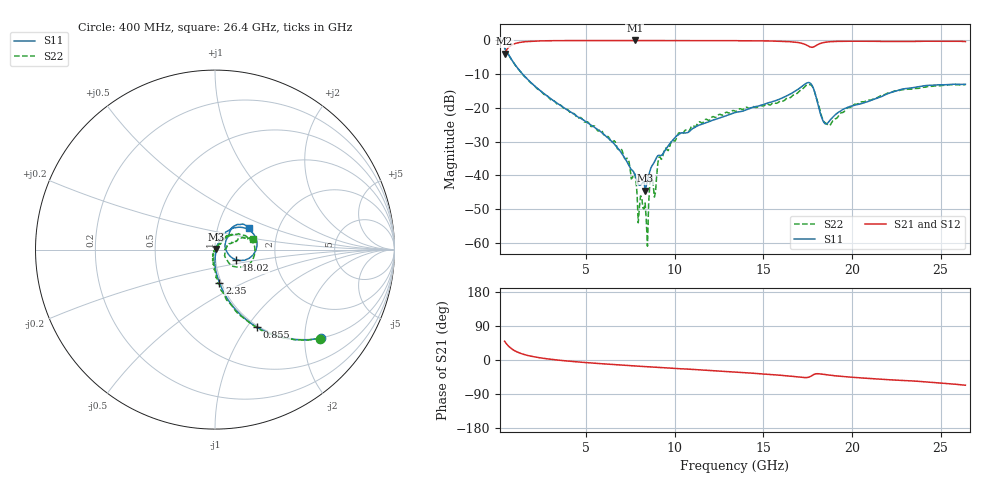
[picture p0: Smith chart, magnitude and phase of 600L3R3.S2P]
!  American Technical Ceramics  Date:  10/27/06
!  One Norden Lane
!  Huntington Station,  NY.  11746-2102
!  Tel:  (631) 622-4700  Fax:  (631) 622-4748
!  Part Number  600L3R3		Mounting Orientation: Vertical
!  Description: Ultra Low ESR Microwave capacitors
!  Application: Coupling, Bypass, Tuning, DC Block
!  Filters, Matching
# GHZ S DB R 50
! Freq  |S11|  S11 Ph  |S21|  S21 Ph  |S12|  S12 Ph  |S22|  S22 Ph
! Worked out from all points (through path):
!   401 points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, 400 MHz to 26.4 GHz, reference 50 ohm
!   highest |S21| = -0.02 dB at 7.745 GHz (marker M1); lowest = -4.0 dB at 400 MHz (marker M2)
!   group delay of S21, straight-line fit = 8.26 ps
!   lowest |S11| = -44.5 dB at 8.33 GHz (marker M3), VSWR 1.01, Z = 50.5 + j0.282 ohm
!   |S11| at or under -10 dB: 1.42 GHz to end of sweep
!   |S22| runs from -60.9 to -2.3 dB; largest |S21 - S12| = 0.0024
!   S11 on the Smith chart (normalised r, x): 400 MHz: 0.99, -2.40; 855 MHz: 0.98, -1.12; 2.35 GHz: 0.98, -0.37; 18.02 GHz: 1.26, -0.15; 26.4 GHz: 1.41, +0.36
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0.4  -2.27 -39.9  -3.96 49.4  -3.97 49.5  -2.31 -40.3
0.855  -6.18 -61.6  -1.23 27.7  -1.24 27.7  -6.21 -62.2
2.35  -14.63 -82.4  -0.16 6.1  -0.17 6.2  -14.64 -85.5
4.755  -23.26 -90.3  -0.04 -6.0  -0.04 -6.0  -23.10 -97.4
6.64  -31.01 -84.4  -0.03 -12.3  -0.03 -12.3  -30.03 -109.5
7.745  -39.59 -48.8  -0.02 -15.6  -0.02 -15.6  -39.58 -118.4
7.94  -42.60 -29.9  -0.03 -16.3  -0.03 -16.3  -54.01 -107.3
8.2  -42.10 12.8  -0.04 -17.1  -0.04 -17.1  -49.57 -62.0
8.33  -44.53 28.1  -0.04 -17.4  -0.04 -17.4  -48.14 19.0
8.525  -40.00 47.0  -0.05 -18.0  -0.05 -17.9  -48.66 -12.3
8.655  -37.77 49.6  -0.05 -18.3  -0.05 -18.3  -39.75 25.1
8.915  -35.33 51.4  -0.06 -19.0  -0.06 -19.0  -44.96 36.5
9.11  -34.02 48.8  -0.05 -19.4  -0.05 -19.4  -34.57 66.5
10.28  -27.65 60.1  -0.06 -23.0  -0.05 -23.0  -27.34 54.4
13.4  -21.39 63.3  -0.09 -31.9  -0.08 -31.9  -20.95 51.3
16.975  -14.42 40.8  -0.64 -44.8  -0.63 -44.7  -15.34 28.0
17.755  -13.38 -8.1  -2.05 -40.8  -2.03 -40.8  -13.56 -21.9
18.015  -17.60 -25.7  -1.39 -36.2  -1.38 -36.2  -17.34 -43.1
18.34  -23.47 -10.2  -0.71 -37.5  -0.70 -37.5  -23.27 -35.8
18.665  -24.27 24.1  -0.43 -39.5  -0.43 -39.6  -25.11 -3.8
22.11  -15.60 51.3  -0.34 -52.1  -0.33 -52.2  -15.45 23.7
26.4  -13.00 32.6  -0.35 -66.5  -0.34 -66.6  -13.16 15.7
